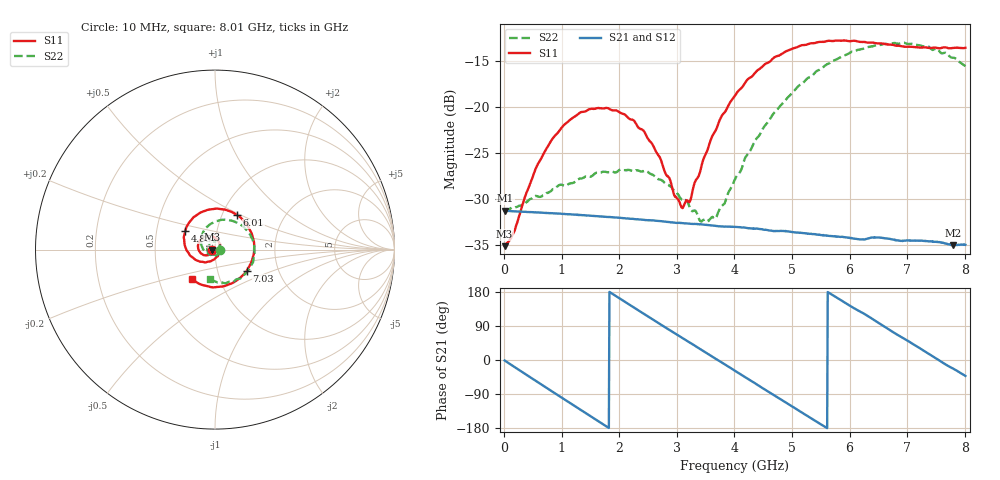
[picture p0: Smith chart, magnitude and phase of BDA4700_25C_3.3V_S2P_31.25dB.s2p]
!Agilent Technologies,E5071B,MY42404982,A.09.10
!Date: Mon Oct 20 18:16:13 2025
!Data & Calibration Information:
!Freq	S11:SOLT2(ON)	S21:SOLT2(ON)	S12:SOLT2(ON)	S22:SOLT2(ON)
# Hz S RI R 50
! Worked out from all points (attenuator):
!   801 points, 10 MHz to 8.01 GHz, reference 50 ohm
!   highest |S21| = -31.29 dB at 20 MHz (marker M1); lowest = -35.1 dB at 7.79 GHz (marker M2)
!   lowest |S11| = -35.2 dB at 10 MHz (marker M3), VSWR 1.04, Z = 48.3 - j0.0936 ohm
!   |S11| at or under -10 dB: start of sweep to end of sweep
!   |S22| runs from -32.5 to -13.0 dB; largest |S21 - S12| = 0.00031
!   S11 on the Smith chart (normalised r, x): 10 MHz: 0.97, -0.00; 4.85 GHz: 0.70, +0.16; 6.01 GHz: 1.18, +0.48; 7.03 GHz: 1.38, -0.34; 8.01 GHz: 0.73, -0.25
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1e7  -0.0174 -0.000969  0.0272 -0.000591  0.0272 -0.000611  0.0272 -0.000814
2e7  -0.0178 -0.00158  0.0272 -0.00103  0.0272 -0.00108  0.0271 -0.00106
1.6e8  -0.0182 -0.00946  0.026 -0.00761  0.026 -0.00759  0.0273 -0.00771
5.4e8  -0.035 -0.0288  0.0157 -0.0216  0.0157 -0.0216  0.0164 -0.0283
7.3e8  -0.0494 -0.032  0.00789 -0.0253  0.0079 -0.0253  0.00419 -0.0336
1.35e9  -0.0937 0.00303  -0.0178 -0.0187  -0.0178 -0.0187  -0.0364 -0.0183
2.08e9  -0.0552 0.0729  -0.0226 0.0103  -0.0226 0.0104  -0.0303 0.0336
2.42e9  -0.0121 0.0733  -0.0131 0.0205  -0.0131 0.0205  -0.00538 0.0443
2.68e9  0.0159 0.0521  -0.00319 0.0237  -0.00319 0.0237  0.0126 0.0384
3.11e9  0.0277 -0.00667  0.0128 0.0195  0.0127 0.0195  0.0288 0.0112
3.23e9  0.0216 -0.022  0.0162 0.0165  0.0162 0.0165  0.028 0.00301
3.55e9  -0.0137 -0.059  0.022 0.00589  0.022 0.00583  0.0132 -0.02
3.7e9  -0.0389 -0.0672  0.0225 0.000331  0.0225 0.000273  0.000546 -0.0257
4.01e9  -0.0969 -0.0617  0.0196 -0.0106  0.0196 -0.0105  -0.0309 -0.0259
4.85e9  -0.1651 0.1061  -0.0066 -0.0201  -0.0064 -0.0201  -0.0751 0.0739
5.35e9  -0.0749 0.2087  -0.0185 -0.00839  -0.0185 -0.00856  -0.0162 0.1465
6.01e9  0.1235 0.1912  -0.0154 0.0117  -0.0156 0.0116  0.1327 0.1462
6.68e9  0.2178 -0.00272  0.0032 0.0189  0.00321 0.0189  0.2187 0.00105
7.03e9  0.1774 -0.1169  0.0124 0.0141  0.0125 0.014  0.199 -0.0928
7.45e9  0.0572 -0.2018  0.0183 0.00289  0.0183 0.00286  0.1137 -0.1701
7.79e9  -0.0632 -0.1991  0.0163 -0.00662  0.0163 -0.00677  0.0233 -0.1834
8.01e9  -0.1307 -0.1637  0.0132 -0.0119  0.0132 -0.0119  -0.0296 -0.1635
